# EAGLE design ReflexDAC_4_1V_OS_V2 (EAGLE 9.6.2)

## Sheet 1 of 3: Analog Circuits
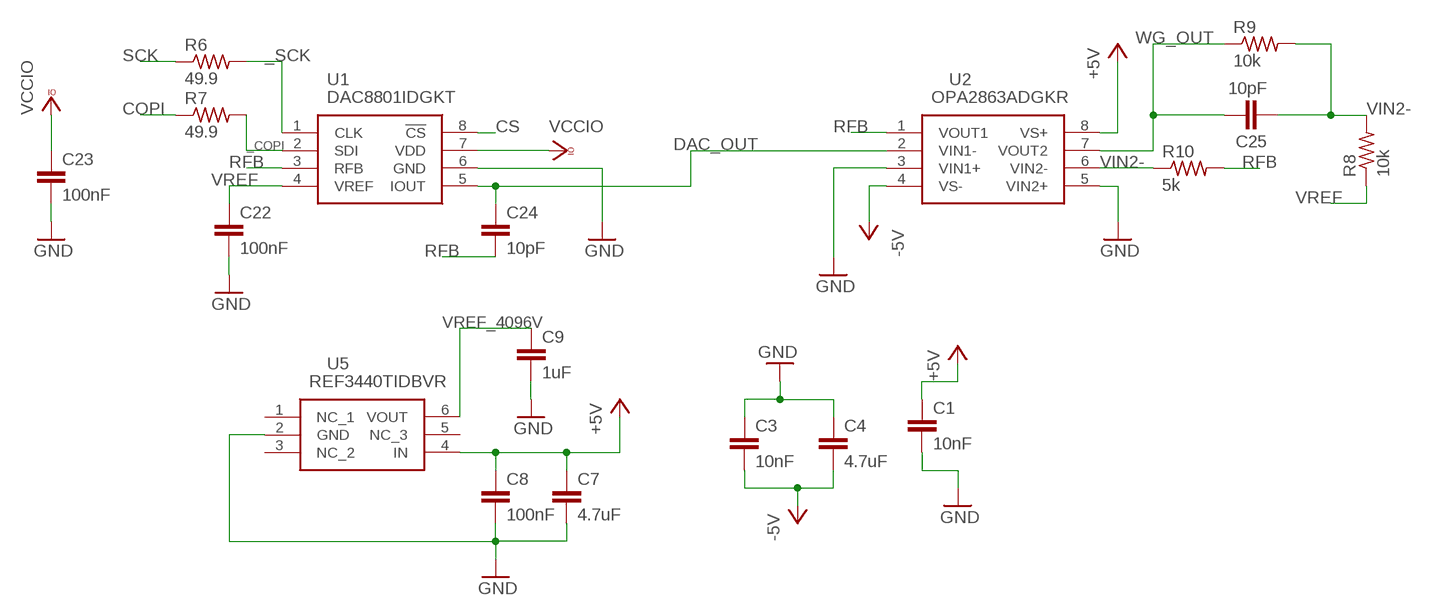
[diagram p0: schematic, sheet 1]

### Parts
C1  10nF  C-EUC0603  [C0603]
C3  10nF  C-EUC0603  [C0603]
C4  4.7uF  C-EUC0603  [C0603]
C7  4.7uF  C-EUC0603  [C0603]
C8  100nF  C-EUC0603  [C0603]
C9  1uF  C-EUC0603  [C0603]
C22  100nF  C-EUC0603  [C0603]
C23  100nF  C-EUC0603  [C0603]
C24  10pF  C-EUC0603  [C0603]
C25  10pF  C-EUC0603  [C0603]
R6  49.9  R-US_R0603  [R0603]
R7  49.9  R-US_R0603  [R0603]
R8  10k  R-US_R0603  [R0603]
R9  10k  R-US_R0603  [R0603]
R10  5k  R-US_R0603  [R0603]
U1  DAC8801IDGKT  [SOP65P490X110-8N]
U2  OPA2863ADGKR  [SOP65P490X110-8N]
U5  REF3440TIDBVR  [SOT95P280X145-6N]

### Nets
+5V: C1.1 C7.1 C8.1 U2.8(VS+) U5.4(IN) ; also sheet 2,3
-5V: C3.2 C4.2 U2.4(VS-) ; also sheet 2
_COPI: R7.2 U1.2(SDI)
_SCK: R6.2 U1.1(CLK)
COPI: R7.1 ; also sheet 3
CS: U1.8(!CS) ; also sheet 3
DAC_OUT: C24.1 U1.5(IOUT) U2.2(VIN1-)
GND: C1.2 C3.1 C4.1 C7.2 C8.2 C9.2 C22.2 C23.2 U1.6(GND) U2.3(VIN1+) U2.5(VIN2+) U5.2(GND) ; also sheet 2,3
RFB: C24.2 R10.2 U1.3(RFB) U2.1(VOUT1)
SCK: R6.1 ; also sheet 3
VCCIO: C23.1 U1.7(VDD) ; also sheet 2,3
VIN2-: C25.2 R8.2 R9.2 R10.1 U2.6(VIN2-)
VREF: C22.1 R8.1 U1.4(VREF) ; also sheet 3
VREF_4096V: C9.1 U5.6(VOUT) ; also sheet 3
WG_OUT: C25.1 R9.1 U2.7(VOUT2) ; also sheet 3
Unconnected: U5.1(NC_1) U5.3(NC_2) U5.5(NC_3)

## Sheet 2 of 3: Power Circuits
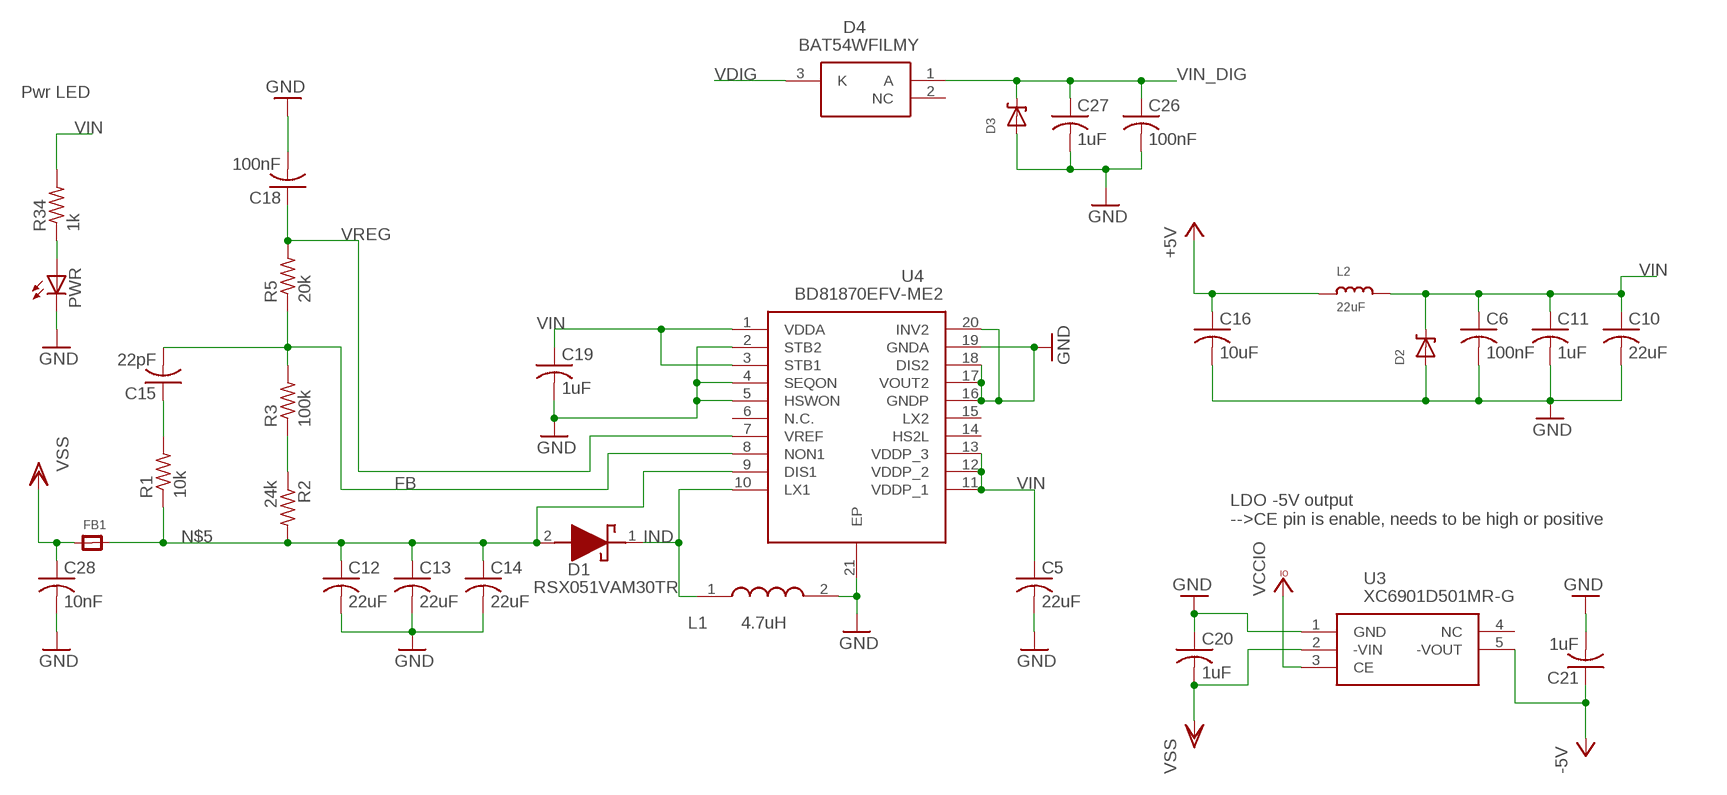
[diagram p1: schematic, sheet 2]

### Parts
C5  22uF  C-USC0603  [C0603]
C6  100nF  C-USC0603  [C0603]
C10  22uF  C-USC0603  [C0603]
C11  1uF  C-USC0603  [C0603]
C12  22uF  C-USC0603  [C0603]
C13  22uF  C-USC0603  [C0603]
C14  22uF  C-USC0603  [C0603]
C15  22pF  C-USC0603  [C0603]
C16  10uF  C-USC0603  [C0603]
C18  100nF  C-USC0603  [C0603]
C19  1uF  C-USC0603  [C0603]
C20  1uF  C-USC0603  [C0603]
C21  1uF  C-USC0603  [C0603]
C26  100nF  C-USC0603  [C0603]
C27  1uF  C-USC0603  [C0603]
C28  10nF  C-USC0603  [C0603]
D1  RSX051VAM30TR  [RSX051VAM30TR]
D2  DDZ5V6ASF  [DDZ5V6ASF]
D3  DDZ5V6ASF  [DDZ5V6ASF]
D4  BAT54WFILMY  [SOT65P210X110-3N]
FB1  FERRITE  [0603]
L1  4.7uH  LQM21PN4R7MGSD  [LQM21PHR47NG0D]
L2  22uF  INDUCTOR0805  [0805]
PWR  LEDCHIPLED_0603  [CHIPLED_0603]
R1  10k  R-US_R0603  [R0603]
R2  24k  R-US_R0603  [R0603]
R3  100k  R-US_R0603  [R0603]
R5  20k  R-US_R0603  [R0603]
R34  1k  R-US_R0603  [R0603]
U3  XC6901D501MR-G  [SOT95P280X130-5N]
U4  BD81870EFV-ME2  [SOP65P640X100-21N]

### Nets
+5V: C16.1 L2.1 ; also sheet 1,3
-5V: C21.1 U3.5(-VOUT) ; also sheet 1
FB: C15.2 R3.2 R5.1 U4.8(NON1)
GND: C5.2 C6.2 C10.2 C11.2 C12.2 C13.2 C14.2 C16.2 C18.2 C19.2 C20.1 C21.2 C26.2 C27.2 C28.2 D2.P$1(A) D3.P$1(A) L1.2 PWR.C U3.1(GND) U4.2(STB2) U4.4(SEQON) U4.5(HSWON) U4.16(GNDP) U4.17(VOUT2) U4.18(DIS2) U4.19(GNDA) U4.20(INV2) U4.21(EP) ; also sheet 1,3
IND: D1.1(K) L1.1 U4.10(LX1)
N$5: C12.1 C13.1 C14.1 D1.2(A) FB1.2 R1.1 R2.2 U4.9(DIS1)
N$7: C15.1 R1.2
N$10: R2.1 R3.1
N$19: PWR.A R34.1
VCCIO: U3.3(CE) ; also sheet 1,3
VDIG: D4.3(K) ; also sheet 3
VIN: C5.1 C6.1 C10.1 C11.1 C19.1 D2.P$2(C) L2.2 R34.2 U4.1(VDDA) U4.3(STB1) U4.11(VDDP_1) U4.12(VDDP_2) U4.13(VDDP_3) ; also sheet 3
VIN_DIG: C26.1 C27.1 D3.P$2(C) D4.1(A) ; also sheet 3
VREG: C18.1 R5.2 U4.7(VREF)
VSS: C20.2 C28.1 FB1.1 U3.2(-VIN)
Unconnected: D4.2(NC) U3.4(NC) U4.6(N.C.) U4.14(HS2L) U4.15(LX2)

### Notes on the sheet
- Pwr LED
- LDO -5V output
  -->CE pin is enable, needs to be high or positive

## Sheet 3 of 3: Connectors and analog switch
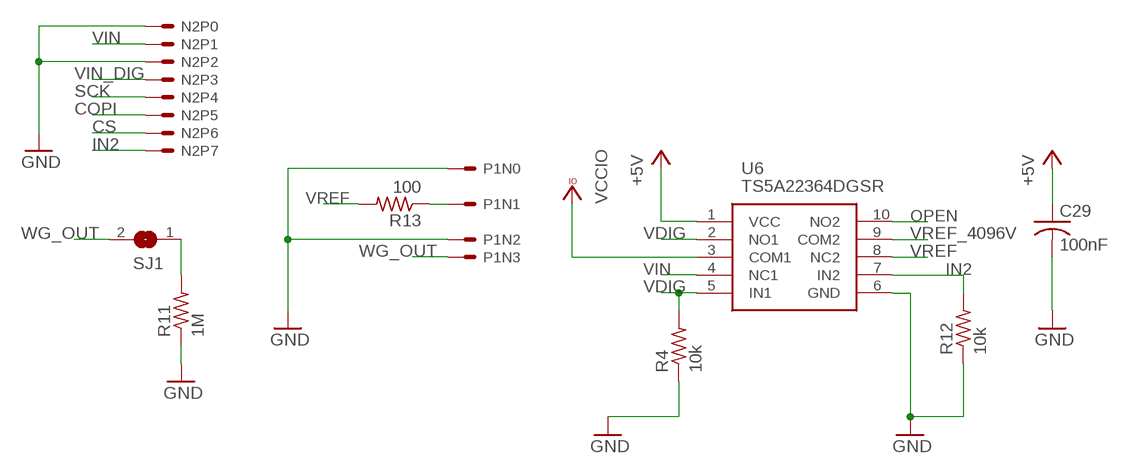
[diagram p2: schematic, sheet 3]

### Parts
C29  100nF  C-USC0603  [C0603]
N2  8PINHEADER  [8PINHEADER]
P1  4PINHEADER  [4PINHEADER]
R4  10k  R-US_R0603  [R0603]
R11  1M  R-US_R0603  [R0603]
R12  10k  R-US_R0603  [R0603]
R13  100  R-US_R0603  [R0603]
SJ1  SOLDERJUMPER  [SOLDERJUMPER_ARROW_NOPASTE]
U6  TS5A22364DGSR  [SOP50P490X110-10N]

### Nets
+5V: C29.1 U6.1(VCC) ; also sheet 1,2
COPI: N2.P5 ; also sheet 1
CS: N2.P6 ; also sheet 1
GND: C29.2 N2.P0 N2.P2 P1.N0 P1.N2 R4.1 R11.1 R12.1 U6.6(GND) ; also sheet 1,2
IN2: N2.P7 R12.2 U6.7(IN2)
N$1: R11.2 SJ1.1
N$2: P1.N1 R13.1
OPEN: U6.10(NO2)
SCK: N2.P4 ; also sheet 1
VCCIO: U6.3(COM1) ; also sheet 1,2
VDIG: R4.2 U6.2(NO1) U6.5(IN1) ; also sheet 2
VIN: N2.P1 U6.4(NC1) ; also sheet 2
VIN_DIG: N2.P3 ; also sheet 2
VREF: R13.2 U6.8(NC2) ; also sheet 1
VREF_4096V: U6.9(COM2) ; also sheet 1
WG_OUT: P1.N3 SJ1.2 ; also sheet 1

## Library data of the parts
C1 C3 C4 C7-C9 C22-C25 = rcl:C-EU: CAPACITOR, European symbol; SPICEPREFIX: C
C5 C6 C10-C16 C18-C21 C26-C29 = rcl:C-US: CAPACITOR, American symbol; SPICEPREFIX: C
D1 = SamacSys_Parts:RSX051VAM30TR: ROHM 30V 500mA, SiC Schottky Diode, 2-Pin SOD-323HE RSX051VAM30TR; DESCRIPTION: ROHM 30V 500mA, SiC Schottky Diode, 2-Pin SOD-323HE RSX051VAM30TR; HEIGHT: 0.8mm; MANUFACTURER_NAME: ROHM Semiconductor; MANUFACTURER_PART_NUMBER: RSX051VAM30TR; MOUSER_PART_NUMBER: 755-RSX051VAM30TR; MOUSER_PRICE-STOCK: https://www.mouser.co.uk/ProductDetail/ROHM-Semiconductor/RSX051VAM30TR?qs=4v%252BiZTmLVHH6gyykIHF0SA%3D%3D
D2 D3 = ForceTronics:DDZ5V6ASF: DDZ5V6ASF 5.42 Zener Diode
D4 = SamacSys_Parts:BAT54WFILMY: Automotive 40 V, 300 mA General purpose Small Signal Schottky Diode Source: Datasheet; DESCRIPTION: Automotive 40 V, 300 mA General purpose Small Signal Schottky Diode; HEIGHT: 1.1mm; MANUFACTURER_NAME: STMicroelectronics; MANUFACTURER_PART_NUMBER: BAT54WFILMY; MOUSER_PART_NUMBER: 511-BAT54WFILMY; MOUSER_PRICE-STOCK: https://www.mouser.co.uk/ProductDetail/STMicroelectronics/BAT54WFILMY?qs=aA7MvVR8Lz8Zb51n0tQT7w%3D%3D
FB1 = microbuilder:FERRITE: Ferrite Bead
L1 = SamacSys_Parts:LQM21PN4R7MGSD: LQM21PN_GS Series Inductor 4.7uH +/-20% 0805 (2012); DESCRIPTION: LQM21PN_GS Series Inductor 4.7uH +/-20% 0805 (2012); HEIGHT: 1mm; MANUFACTURER_NAME: Murata Electronics; MANUFACTURER_PART_NUMBER: LQM21PN4R7MGSD; MOUSER_PART_NUMBER: 81-LQM21PN4R7MGSD; MOUSER_PRICE-STOCK: https://www.mouser.co.uk/ProductDetail/Murata-Electronics/LQM21PN4R7MGSD?qs=Gufeu08L%2Fl2uzbzo%2FrY4bg%3D%3D
L2 = microbuilder:INDUCTOR: Inductors
N2 = ForceTronics:8PINHEADER: 8 pin header with 2.54mm spacing
P1 = ForceTronics:4PINHEADER
PWR = adafruit:LED: LED
R1-R13 R34 = rcl:R-US_: RESISTOR, American symbol; SPICEPREFIX: R
SJ1 = microbuilder:SOLDERJUMPER: SMD Solder JUMPER; BOM: EXCLUDE
U1 = SamacSys_Parts:DAC8801IDGKT: 14-Bit, Single Channel, Serial Interface, Multiplying Digital-to-Analog Converter Source: Datasheet; DESCRIPTION: 14-Bit, Single Channel, Serial Interface, Multiplying Digital-to-Analog Converter; HEIGHT: 1.1mm; MANUFACTURER_NAME: Texas Instruments; MANUFACTURER_PART_NUMBER: DAC8801IDGKT; MOUSER_PART_NUMBER: 595-DAC8801IDGKT; MOUSER_PRICE-STOCK: https://www.mouser.co.uk/ProductDetail/Texas-Instruments/DAC8801IDGKT?qs=vul0MlC%2Fa1fY4dNbzQeDsA%3D%3D
U2 = SamacSys_Parts:OPA2863ADGKR: Precision Amplifiers Dual, high-precision, low-power, 105MHz, 12V RRIO voltage-feedback amplifier Source: Datasheet; DESCRIPTION: Precision Amplifiers Dual, high-precision, low-power, 105MHz, 12V RRIO voltage-feedback amplifier; HEIGHT: 1.1mm; MANUFACTURER_NAME: Texas Instruments; MANUFACTURER_PART_NUMBER: OPA2863ADGKR
U3 = SamacSys_Parts:XC6901D501MR-G: LDO Voltage Regulators Source: Datasheet; DESCRIPTION: LDO Voltage Regulators; HEIGHT: 1.3mm; MANUFACTURER_NAME: Torex; MANUFACTURER_PART_NUMBER: XC6901D501MR-G; MOUSER_PART_NUMBER: 865-XC6901D501MR-G; MOUSER_PRICE-STOCK: https://www.mouser.co.uk/ProductDetail/Torex-Semiconductor/XC6901D501MR-G?qs=AsjdqWjXhJ83wf2WZneG3A%3D%3D
U4 = SamacSys_Parts:BD81870EFV-ME2: ROHM - BD81870EFV-ME2 - DC/DC Switching Regulator, Inverting, Step Up, 2 Output, 2.5V to 5.5VIn, 18V out, 2.1MHz, HTSSOP-20 Source: Datasheet; DESCRIPTION: ROHM - BD81870EFV-ME2 - DC/DC Switching Regulator, Inverting, Step Up, 2 Output, 2.5V to 5.5VIn, 18V out, 2.1MHz, HTSSOP-20; HEIGHT: 1mm; MANUFACTURER_NAME: ROHM Semiconductor; MANUFACTURER_PART_NUMBER: BD81870EFV-ME2; MOUSER_PART_NUMBER: 755-BD81870EFV-ME2; MOUSER_PRICE-STOCK: https://www.mouser.co.uk/ProductDetail/ROHM-Semiconductor/BD81870EFV-ME2/?qs=HXFqYaX1Q2wm5IkeUd4YKg%3D%3D
U5 = SamacSys_Parts:REF3440TIDBVR: Voltage References 4.1-V, low-drift, low-power, small-footprint series voltage reference Source: Datasheet; DESCRIPTION: Voltage References 4.1-V, low-drift, low-power, small-footprint series voltage reference; HEIGHT: 1.45mm; MANUFACTURER_NAME: Texas Instruments; MANUFACTURER_PART_NUMBER: REF3440TIDBVR; MOUSER_PART_NUMBER: 595-REF3440TIDBVR; MOUSER_PRICE-STOCK: https://www.mouser.co.uk/ProductDetail/Texas-Instruments/REF3440TIDBVR?qs=aP1CjGhiNiFrJEFwygVNiw%3D%3D
U6 = SamacSys_Parts:TS5A22364DGSR: Analog Switch ICs 0.65-Ohm Dual SPDT Analog Switch Source: Datasheet; DESCRIPTION: Analog Switch ICs 0.65-Ohm Dual SPDT Analog Switch; HEIGHT: 1.1mm; MANUFACTURER_NAME: Texas Instruments; MANUFACTURER_PART_NUMBER: TS5A22364DGSR; MOUSER_PART_NUMBER: 595-TS5A22364DGSR; MOUSER_PRICE-STOCK: https://www.mouser.co.uk/ProductDetail/Texas-Instruments/TS5A22364DGSR?qs=9F2IyUQaA%2FhbjQmUI4VB%2FQ%3D%3D

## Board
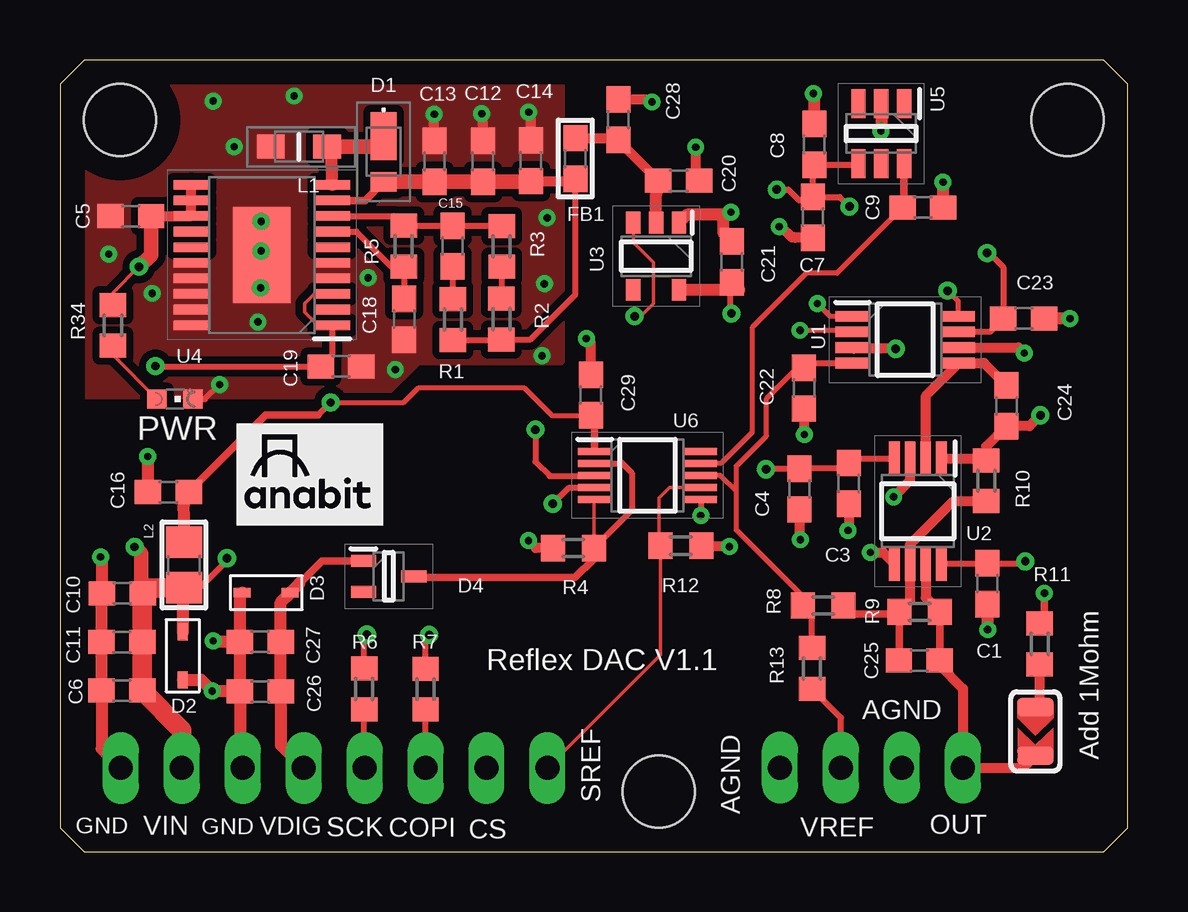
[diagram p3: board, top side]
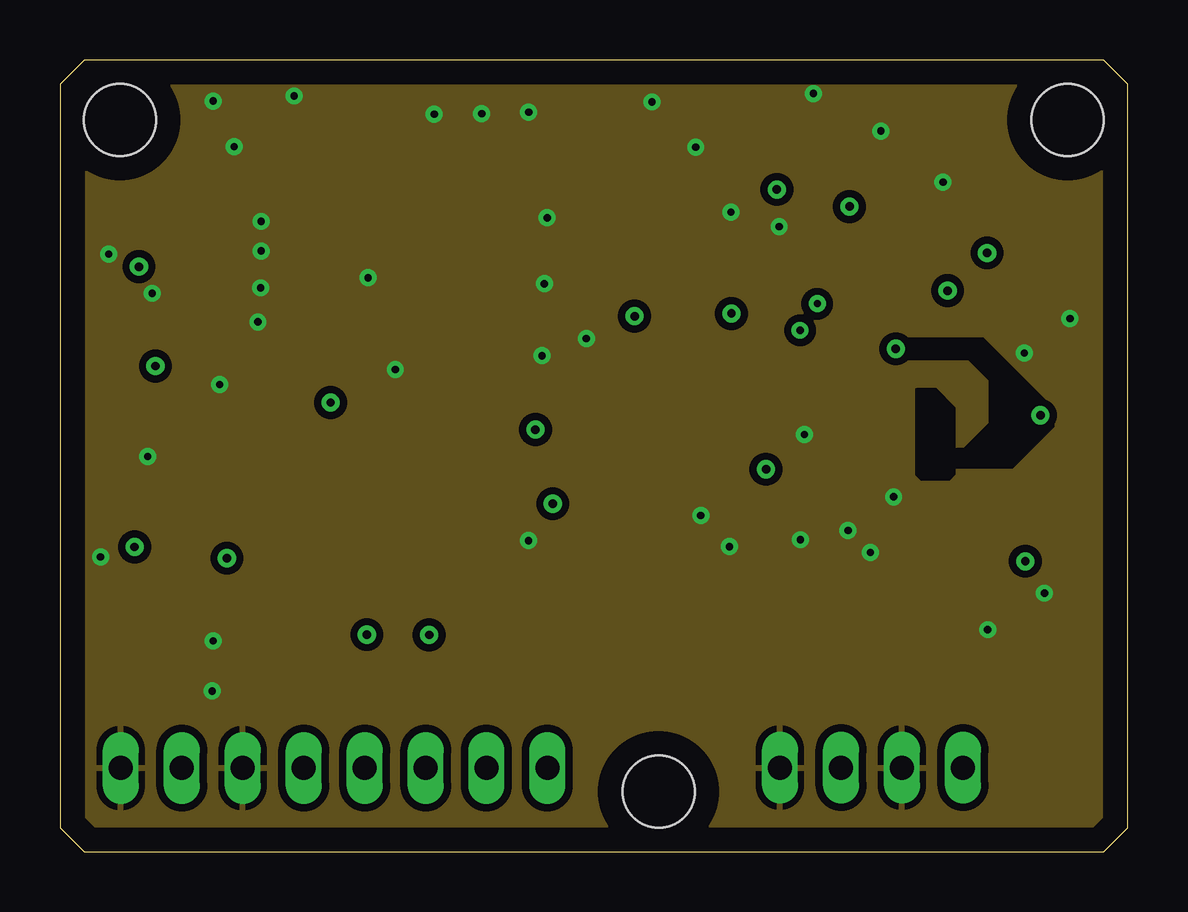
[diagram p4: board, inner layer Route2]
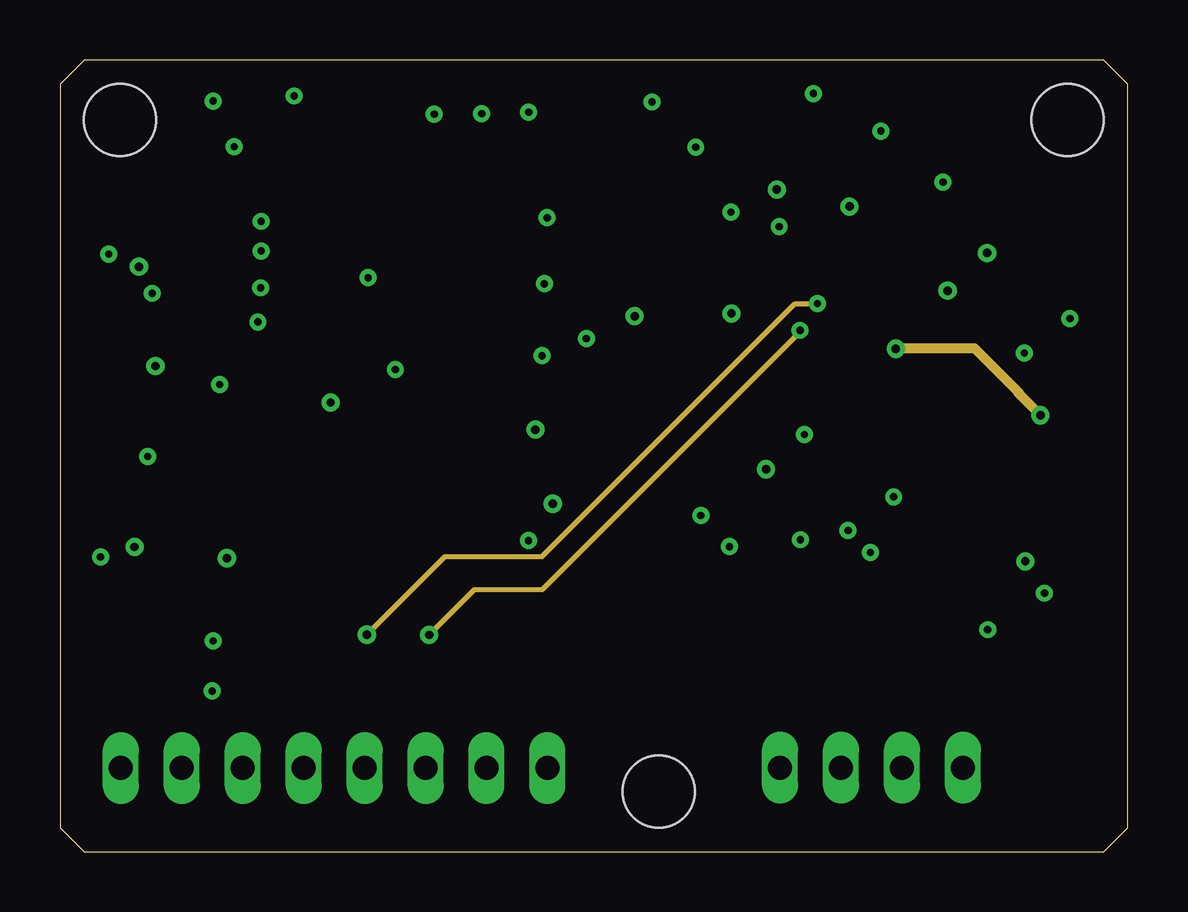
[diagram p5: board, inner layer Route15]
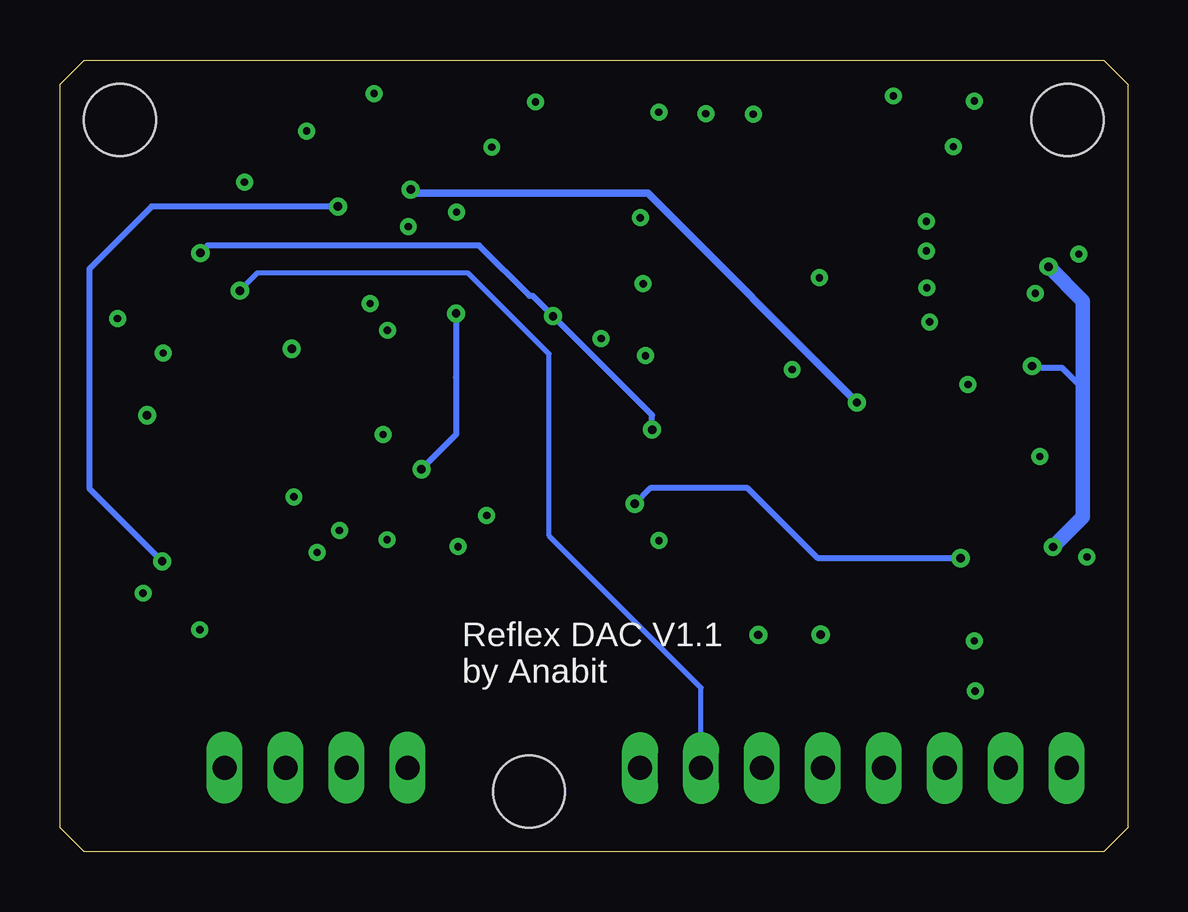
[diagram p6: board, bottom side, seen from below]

Size 44.5 x 33 mm. Coordinates in mm from the lower left corner, seen from the top.
Outline: 0,32 0,1 1,0 43.5,0 44.5,1 44.5,32 43.5,33 1,33 0,32
Copper layers (1+2*15+16): Top 0.035mm / dielectric 0.5mm / Route2 0.035mm / dielectric 0.6mm / Route15 0.035mm / dielectric 0.5mm / Bottom 0.035mm
Design rules "default *": minimum track width 6mil, minimum drill 0.3mm, track to track 6mil, track to pad 6mil, pad to pad 6mil, via to via 6mil, smd to smd 6mil, copper to edge 40mil, drill to drill 6mil, minimum pad ring 10mil, minimum via ring 8mil, stop-mask expansion 4mil, vias tented up to drill 0mil, thermal gap 10mil
Holes 3 mm at 2.5,30.5 24.95,2.5 42,30.5

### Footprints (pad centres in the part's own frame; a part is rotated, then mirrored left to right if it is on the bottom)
C0603 = smd 1.1 x 1: 1 -0.85,0; 2 0.85,0
RSX051VAM30TR = smd 1.1 x 2: 1 0,0.65 | smd 1.1 x 0.8: 2 0,-1.25
DDZ5V6ASF = smd 0.71 x 0.41: P$1 0,0; P$2 1.99,0
SOT65P210X110-3N = smd 1.05 x 0.5: 1 -1.05,0.65; 2 -1.05,-0.65; 3 1.05,0
0603 = smd 1.1 x 1: 1 -0.85,0; 2 0.85,0
LQM21PHR47NG0D = smd 1.15 x 1: 1 -1.175,0; 2 1.175,0
0805 = smd 1.3 x 1.5: 1 -0.95,0; 2 0.95,0
8PINHEADER = drill 1 long: P0 1.27,-3.81; P1 3.81,-3.81; P2 6.35,-3.81; P3 8.89,-3.81; P4 11.43,-3.81; P5 13.97,-3.81; P6 16.51,-3.81; P7 19.05,-3.81
4PINHEADER = drill 1 long: N0 -3.81,0; N1 -1.27,0; N2 1.27,0; N3 3.81,0
CHIPLED_0603 = smd 0.8 x 0.8: A 0,-0.75; C 0,0.75
R0603 = smd 1 x 1.1: 1 -0.85,0; 2 0.85,0
SOLDERJUMPER_ARROW_NOPASTE = smd 0.762 x 1.524: 1 -1.016,0; 2 1.016,0
SOP65P490X110-8N = smd 1.4 x 0.45: 1 -2.2,0.975; 2 -2.2,0.325; 3 -2.2,-0.325; 4 -2.2,-0.975; 5 2.2,-0.975; 6 2.2,-0.325; 7 2.2,0.325; 8 2.2,0.975
SOT95P280X130-5N = smd 0.9 x 0.6: 1 -1.4,0.95; 2 -1.4,0; 3 -1.4,-0.95; 4 1.4,-0.95; 5 1.4,0.95
SOP65P640X100-21N = smd 1.475 x 0.4: 1 -2.938,2.925; 2 -2.938,2.275; 3 -2.938,1.625; 4 -2.938,0.975; 5 -2.938,0.325; 6 -2.938,-0.325; 7 -2.938,-0.975; 8 -2.938,-1.625; 9 -2.938,-2.275; 10 -2.938,-2.925; 11 2.938,-2.925; 12 2.938,-2.275; 13 2.938,-1.625; 14 2.938,-0.975; 15 2.938,-0.325; 16 2.938,0.325; 17 2.938,0.975; 18 2.938,1.625; 19 2.938,2.275; 20 2.938,2.925 | smd 2.4 x 4: 21 0,0
SOT95P280X145-6N = smd 1.2 x 0.6: 1 -1.25,0.95; 2 -1.25,0; 3 -1.25,-0.95; 4 1.25,-0.95; 5 1.25,0; 6 1.25,0.95
SOP50P490X110-10N = smd 1.4 x 0.3: 1 -2.2,1; 2 -2.2,0.5; 3 -2.2,0; 4 -2.2,-0.5; 5 -2.2,-1; 6 2.2,-1; 7 2.2,-0.5; 8 2.2,0; 9 2.2,0.5; 10 2.2,1

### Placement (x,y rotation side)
C1  38.65,11.17 270 top
C3  32.88,15.35 90 top
C4  30.83,15.11 90 top
C5  2.95,26.49 180 top
C6  2.58,6.71 180 top
C7  31.38,26.44 270 top
C8  31.44,29.48 90 top
C9  35.97,26.84 0 top
C10  2.6,10.77 180 top
C11  2.58,8.74 180 top
C12  17.63,28.77 90 top
C13  15.62,28.77 90 top
C14  19.63,28.8 90 top
C15  16.37,25.24 90 top
C16  4.52,14.99 180 top
C18  14.34,22.19 270 top
C19  11.72,20.22 0 top
C20  25.79,27.97 180 top
C21  28,24.58 90 top
C22  31.02,19.32 270 top
C23  40.17,22.22 0 top
C24  39.45,18.58 270 top
C25  35.82,7.97 180 top
C26  8.35,6.67 180 top
C27  8.35,8.75 180 top
C28  23.28,30.51 90 top
C29  22.13,19.03 90 top
D1  13.49,29.17 0 top
D2  5.12,7.16 90 top
D3  7.6,10.79 0 top
D4  13.7,11.47 0 top
FB1  21.48,28.89 270 top
L1  9.96,29.38 180 top
L2  5.17,11.95 270 top
N2  1.27,7.29 0 top
P1  33.83,3.5 0 top
PWR  4.79,18.86 270 top
R1  16.38,22.18 90 top
R2  18.4,22.2 270 top
R3  18.41,25.23 90 top
R4  21.4,12.65 0 top
R5  14.33,25.24 270 top
R6  12.68,6.78 90 top
R7  15.24,6.77 90 top
R8  31.81,10.26 0 top
R9  35.83,9.99 180 top
R10  38.61,15.46 90 top
R11  40.84,8.66 270 top
R12  25.88,12.75 180 top
R13  31.35,7.64 90 top
R34  2.21,21.94 90 top
SJ1  40.66,5.01 270 top
U1  35.23,21.34 0 top
U2  35.76,14.19 270 top
U3  24.85,24.82 270 top
U4  8.41,24.87 180 top
U5  34.23,29.93 270 top
U6  24.49,15.68 0 top

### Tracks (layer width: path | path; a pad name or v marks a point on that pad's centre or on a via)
+5V  (via drill 0.35)
  Top 0.2: v11.28,18.72 14.33,18.72 14.95,19.34 19.34,19.34 20.5,18.18 C29.1 22.29,18.02
  Top 0.254: C16.1 5.37,15.25 | 10.76,18.2 v11.28,18.72 | C7.1 31.23,27.14 30.82,27.14 30.36,27.6 v29.88,27.6 | C7.1 31.38,28.57 C8.1 33.23,28.63 U5.4 | C7.1 32.49,27.29 v32.9,26.88 v32.91,26.89 | v40.24,12.1 40.2,12.1 40.12,12.02 C1.1 38.62,11.99 U2.8
  Top 0.305: 10.76,18.2 8.58,18.2 C16.1 | 22.29,18.02 U6.1
  Top 0.508: L2.1 5.17,13.92 5.16,14.44 C16.1
  Bottom 0.254: 29.72,27.44 v29.88,27.6 | v32.91,26.89 40.68,26.89 43.28,24.29 43.28,15.14 v40.24,12.1
  Bottom 0.305: v11.28,18.72 20,27.44 29.72,27.44
-5V  (via drill 0.35)
  Top 0.254: v29.43,15.94 30.57,15.94 30.69,15.82 C4.2 32.64,15.96 C3.2 33.35,16.39 U2.4 | C21.1 27.93,23.66 27.93,22.49 v27.99,22.43
  Top 0.508: U3.5 28.31,23.42 C21.1
  Bottom 0.254: v29.43,15.94 27.98,17.39 27.98,19.77 27.99,19.78 v27.99,22.43
_COPI  (via drill 0.3, 0.35)
  Top 0.2: 30.87,21.71 32.92,21.71 32.88,21.66 U1.2
  Top 0.254: R7.2 15.24,8.9 v15.38,9.04 v15.39,9.03 | v30.85,21.73 30.87,21.71
  Route15 0.2: v15.39,9.03 17.28,10.92 20.11,10.92 30.89,21.7 v30.85,21.73
_SCK  (via drill 0.3, 0.35)
  Top 0.2: v31.57,22.84 32.09,22.32 U1.1
  Top 0.203: R6.2 12.68,7.84
  Top 0.254: R6.2 12.68,8.85 12.83,9 v12.79,9.04
  Route15 0.2: v12.79,9.04 16.05,12.3 20.1,12.3 30.64,22.84 v31.57,22.84
COPI
  Top 0.254: N2.P5 R7.1
CS  (via drill 0.35)
  Top 0.2: v37,23.38 37.43,22.95 U1.8
  Bottom 0.2: N2.P6 17.78,6.83 24.11,13.16 24.11,20.74 27.49,24.12 36.28,24.12 37,23.4 v37,23.38
DAC_OUT
  Top 0.406: U1.5 37.46,20.36 | 37.46,20.36 38.52,20.36 C24.1 | U2.2 36.1,16.41 36.1,19 37.46,20.36
FB
  Top 0.254: U4.8 13.93,26.5 R5.1 C15.2 R3.2
GND  (via drill 0.3)
  Top 0.254: U6.6 26.71,14.66 v26.71,14.01 | PWR.C 6.04,18.86 v6.65,19.47
  Top 0.305: R11.1 41.04,9.71 v41.04,10.77
  Top 0.406: 31.44,31.57 v31.41,31.6 | C4.1 30.83,13.03 v30.86,13 | 27.66,26.35 v27.97,26.66 | C21.2 27.66,25.77 | C7.2 30.65,25.59 30.63,25.61 30.5,25.61 30.06,26.05 v29.98,26.05 | U1.6 39.97,21.02 v40.2,20.78 | U2.3 35.44,15.47 v34.75,14.79 | C3.1 32.88,13.42 v32.85,13.39 | v33.78,12.47 34.3,12.47 U2.5 | C22.2 v31.02,17.4 v31.03,17.39 | C28.2 24.57,31.36 v24.68,31.25 | C20.1 26.5,28.11 v26.5,29.36 | C13.2 15.6,29.64 v15.6,30.74 | C12.2 17.63,30.71 v17.58,30.76 | C14.2 19.63,30.73 v19.54,30.82 | C29.2 22.13,21.2 v21.94,21.39 | R4.1 19.84,12.65 v19.53,12.96 | R12.1 27.87,12.75 v27.91,12.71
  Top 0.508: C8.2 31.44,31.57 | C9.2 v36.82,27.9 v36.81,27.91 | v34.22,30.04 v34.23,30.05 U5.2 | v42.1,22.22 C23.2 | C1.2 38.65,9.27 v38.67,9.25 | v1.69,12.28 1.75,12.22 C10.2 1.73,10.75 C11.2 C6.2 1.73,4.29 N2.P0 | C16.2 v3.67,16.46 v3.66,16.47 | D2.P$1 5.88,7.16 v6.35,6.69 6.37,6.67 C26.2 | C27.2 6.41,8.75 v6.38,8.78 | C27.2 7.5,10.69 D3.P$1 | C26.2 C27.2 | U3.1 26.13,26.55 27.66,26.55 27.66,26.35 27.66,25.77 | C26.2 7.5,3.6 N2.P2
  other vias: 6.38,31.29 2.03,24.91 8.38,26.27 8.38,25.04 8.36,23.5 13.98,20.09 12.84,23.92 3.84,23.27 8.25,22.08 7.26,29.39 9.76,31.5 20.31,26.42 20.19,23.67 20.09,20.67
  pour Top (isolate 0.305, no thermals): 20.3,34 0.5,34 -1,32.5 -1,19.5 -0.4,18.9 13.56,18.9 14.99,20.33 20.93,20.33 21,20.4 21,33.3
  pour Route2 (isolate 0.305): -2,35 46,35 47.5,33.5 47.5,0.5 44.5,-2.5 -0.5,-2.5 -2.5,-0.5 -2.5,34.5
  cutout Route2: 35.7,15.7 35.7,19.3 36.5,19.3 37.29,18.51 37.29,15.72 37.07,15.5 35.9,15.5
  cutout Route2: 35.4,21.4 38.46,21.4 41.4,18.46 41.4,17.7 39.7,16 37.4,16 37.2,16.2 37.2,16.8 37.7,16.8 38.77,17.87 38.77,19.64 37.89,20.52 35.4,20.52
IN2
  Top 0.152: U6.7 25.41,15.18 24.97,14.74 24.97,12.75 R12.2 25.03,8.19 N2.P7
IND
  Top 0.508: U4.10 11.35,28.5 11.3,28.55 11.3,29.21 L1.1 | 13.05,29.38 D1.1
  Top 0.61: L1.1 13.05,29.38
N$1
  Top 0.406: SJ1.1 40.84,6.21 R11.2
N$2
  Top 0.254: P1.N1 32.56,5.58 R13.1
N$5
  Top 0.254: R1.1 18.38,21.33 R2.2 19.61,21.35 21.48,23.22 FB1.2
  Top 0.305: U4.9 12.71,27.14 D1.2
  Top 0.406: C14.1 21.39,27.95 FB1.2
  Top 0.61: D1.2 C13.1 C12.1 19.6,27.92 C14.1
N$7
  Top 0.254: C15.1 R1.2
N$10
  Top 0.254: R3.1 R2.1
N$19
  Top 0.152: R34.1 2.21,20.69 PWR.A
RFB  (via drill 0.35)
  Top 0.305: R10.2 38.45,16.31 38.37,16.39 | 33.09,20.96 U1.3
  Top 0.406: U2.1 38.37,16.39 | v34.84,20.96 33.09,20.96 | v40.87,18.19 40.41,17.73 C24.2 38.61,16.89 R10.2
  Route15 0.406: v34.84,20.96 v34.84,20.97 38.13,20.97 39.96,19.14 39.96,19.1 v40.87,18.19
SCK
  Top 0.254: N2.P4 12.68,3.5 R6.1
VCCIO  (via drill 0.35)
  Top 0.152: v23.95,22.32 24.21,22.32 24.73,22.84 24.73,24.55 23.9,25.38 U3.3
  Top 0.254: 23.86,22.41 v23.95,22.32 | v38.65,24.95 38.73,24.95 39.32,24.37 C23.1 38.77,21.66 U1.7 | 19.82,17.63 v19.82,17.59 19.82,16.25 20.42,15.65 22.26,15.65 U6.3
  Bottom 0.254: v38.65,24.95 38.65,24.98 38.35,25.27 27.03,25.27 24.93,23.17 24.8,23.17 v23.95,22.32 19.82,18.19 v19.82,17.59
VDIG
  Top 0.152: R4.2 22.25,14.64 U6.5
  Top 0.254: R4.2 23.84,14.24 23.84,15.78 23.42,16.2 23.4,16.18 U6.2
  Top 0.305: D4.3 14.8,11.42 21.47,11.42 22.25,12.2 R4.2
VIN  (via drill 0.35)
  Top 0.152: U4.3 10.6,23.25 10.2,22.85 10.2,22.49 10.38,22.31 10.38,22.3 10.74,21.95 U4.1 | v3.29,24.38 2.21,23.3 R34.2
  Top 0.254: U4.1 11.35,20.7 C19.1 4,20.22 v3.98,20.24 | L2.2 5.82,11 7,12.19 v6.96,12.23 | v20.54,14.5 21.19,15.15 22.26,15.15 U6.4
  Top 0.406: C5.1 U4.13 U4.12 U4.11
  Top 0.508: L2.2 5.12,10.95 D2.P$2
  Top 0.61: C10.1 3.39,10.83 3.39,12.42 v3.11,12.7 | C5.1 3.8,24.87 3.31,24.38 v3.29,24.38
  Top 0.813: L2.2 3.68,11 C10.1 3.43,10.75 C11.1 C6.1 5.08,5.06 N2.P1
  Bottom 0.254: 1.86,19.3 2.72,20.16 3.98,20.16 v3.98,20.24 | v6.96,12.23 v6.96,12.24 12.93,12.24 15.84,15.15 19.89,15.15 v20.54,14.5
  Bottom 0.61: v3.11,12.7 1.86,13.95 1.86,19.3 1.86,22.95 v3.29,24.38
VIN2-
  Top 0.305: R9.2 34.98,9.9 | 34.98,9.9 C25.2 | R8.2 33.02,9.9 34.98,9.9
  Top 0.406: R10.1 37.24,14.61 35.44,12.8 U2.6 35.44,10.45 R9.2
VIN_DIG
  Top 0.305: 9.98,11.18 10.92,12.12 D4.1
  Top 0.508: 9.98,11.18 D3.P$2 9.2,10.4 C27.1 C26.1 9.2,4.44 N2.P3
VREF
  Top 0.203: R8.1 30.96,10.64 28.2,13.4 28.2,15.01 | 28.2,15.01 27.52,15.68 U6.8 | 28.2,15.01 28.2,16.07 29.45,17.33 29.45,18.88 30.74,20.17 C22.1
  Top 0.254: R13.2 31.35,9.87 R8.1 | 30.76,20.17 C22.1 31.21,20.36 U1.4
VREF_4096V
  Top 0.203: C9.1 32.39,24.11 31.12,24.11 28.85,21.84 28.85,17.48 27.55,16.18 U6.9
  Top 0.305: U5.6 35.18,26.9 C9.1
VREG
  Top 0.254: U4.7 12.35,25.84 13.8,24.39 R5.2 C18.1
VSS
  Top 0.406: FB1.1 23.2,29.74 C28.1 23.28,29.63 C20.2
  Top 0.508: C20.2 24.85,27.4 U3.2
WG_OUT
  Top 0.305: R9.1 C25.1
  Top 0.406: U2.7 36.09,10.59 R9.1 | C25.1 36.67,7.76 37.64,6.79 P1.N3 40.17,3.5 SJ1.2

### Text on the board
tNames: Reflex DAC V1.1 | AGND | AGND | Add 1Mohm | VIN | SREF | GND | GND | VDIG | SCK | COPI | CS | VREF | OUT
bNames: Reflex DAC V1.1 / by Anabit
